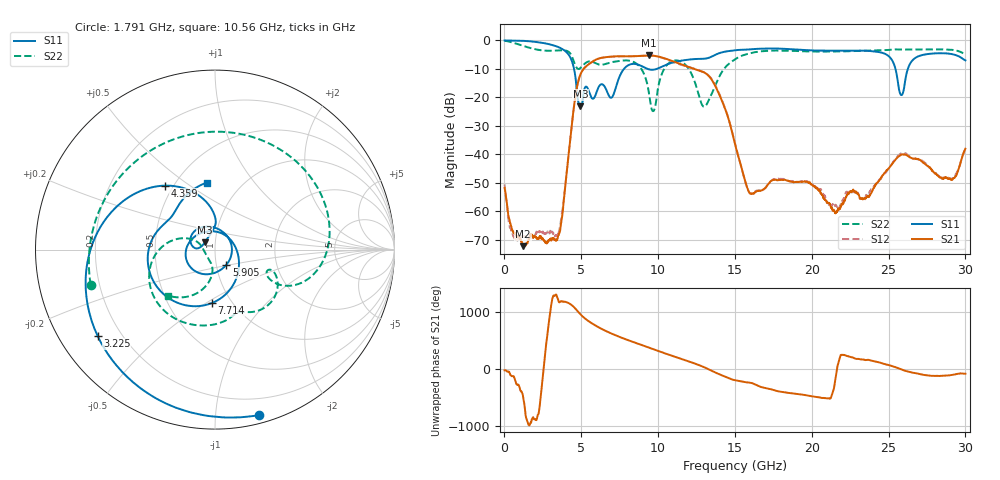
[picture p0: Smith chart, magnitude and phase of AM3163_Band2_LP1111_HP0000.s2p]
!Agilent Technologies,E8364B,MY43040894,A.07.50.67
!Agilent E8364B: A.07.50.67
!Date: Thursday, August 20, 2020 12:02:30
!Correction: S11(Full 2 Port(1,2))
!S21(Full 2 Port(1,2))
!S12(Full 2 Port(1,2))
!S22(Full 2 Port(1,2))
!S2P File: Measurements: S11, S21, S12, S22:
# Hz S  dB  R 50
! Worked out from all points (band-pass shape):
!   3201 points, 10 MHz to 30 GHz, reference 50 ohm
!   highest |S21| = -5.31 dB at 9.391 GHz (marker M1); lowest = -72.3 dB at 1.21 GHz (marker M2)
!   |S21| within 3 dB of the highest: 5.503 GHz to 11.44 GHz (5.935 GHz wide, 70.1 % of centre)
!   lowest |S11| = -23.2 dB at 4.949 GHz (marker M3), VSWR 1.15, Z = 44.6 + j3.61 ohm
!   |S11| at or under -10 dB: 4.528 GHz to 7.784 GHz (3.257 GHz wide, 52.9 % of centre); 9.306 GHz to 9.928 GHz (622 MHz wide, 6.47 % of centre); 25.45 GHz to 26.26 GHz (807.1 MHz wide, 3.12 % of centre)
!   |S22| runs from -24.9 to -0.2 dB; largest |S21 - S12| = 0.013
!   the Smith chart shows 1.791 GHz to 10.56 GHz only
!   S11 on the Smith chart (normalised r, x): 1.791 GHz: 0.06, -1.30; 3.225 GHz: 0.11, -0.32; 4.359 GHz: 0.45, +0.40; 5.905 GHz: 1.12, -0.19; 7.714 GHz: 0.81, -0.53; 10.56 GHz: 0.70, +0.61
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1e7  -0.04 -3.0  -51.91 -26.0  -50.58 57.8  -0.15 -7.1
1.2096e9  -0.17 -50.2  -72.32 -126.7  -68.95 175.2  -1.92 -114.9
1.790656e9  -0.41 -75.2  -68.59 -165.1  -69.28 103.9  -2.86 -164.2
3.224553e9  -1.81 -143.7  -70.02 -151.3  -68.49 -111.4  -3.63 82.3
4.35855e9  -6.86 128.3  -30.88 46.6  -30.87 46.4  -5.29 -17.5
4.948978e9  -23.22 144.2  -11.93 -120.7  -11.93 -120.9  -9.65 -20.0
5.014581e9  -22.91 157.7  -11.17 -138.6  -11.17 -138.9  -9.26 -20.3
5.904909e9  -19.52 -53.4  -6.92 45.7  -6.94 45.5  -7.99 -61.0
6.832725e9  -19.77 95.3  -5.76 -83.1  -5.81 -83.4  -7.89 -83.2
7.713681e9  -10.50 -93.5  -5.58 178.2  -5.63 178.5  -7.08 -115.8
9.391247e9  -10.16 149.7  -5.31 15.1  -5.29 14.9  -18.07 155.7
1.000979e10  -9.82 127.7  -5.68 -45.8  -5.72 -46.5  -16.34 -97.8
1.056273e10  -8.49 96.9  -6.56 -98.8  -6.74 -99.4  -8.75 -135.3
1.300879e10  -6.46 -50.5  -11.31 26.9  -11.26 28.4  -23.34 -102.7
1.5005e10  -3.49 -133.3  -36.40 159.3  -36.35 158.6  -6.68 -112.3
1.597968e10  -3.17 -173.8  -53.71 115.3  -53.83 117.0  -4.55 -171.0
1.786342e10  -2.89 98.0  -49.10 -39.3  -48.72 -39.9  -3.58 92.2
2.000958e10  -3.53 -10.3  -50.76 -124.9  -50.49 -123.2  -3.93 -9.9
2.230569e10  -3.57 -100.3  -54.35 -135.3  -53.41 -140.3  -3.84 -93.6
2.500479e10  -5.54 157.8  -45.01 66.5  -44.85 64.2  -3.36 -167.6
2.583889e10  -19.24 171.2  -40.12 -11.3  -39.66 -8.6  -3.22 169.7
3e10  -7.03 50.6  -38.11 -87.4  -38.29 -84.5  -4.84 54.6
